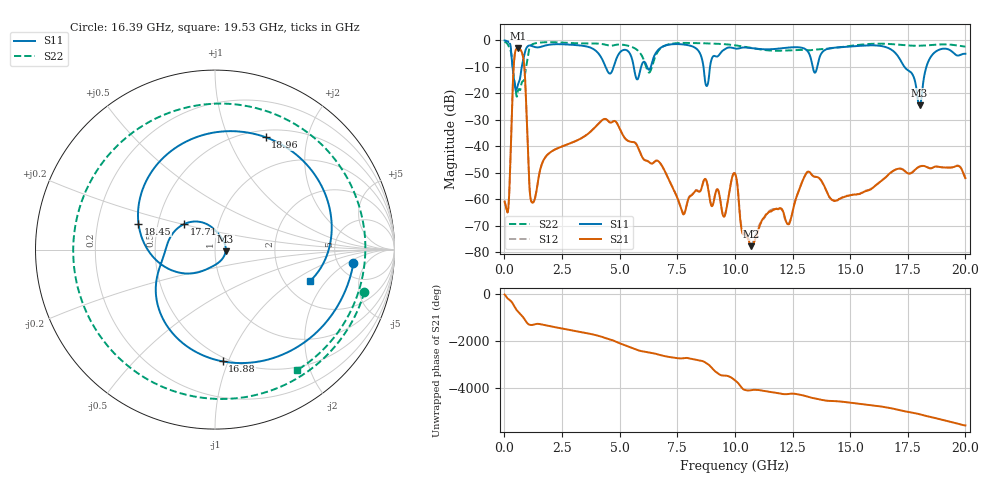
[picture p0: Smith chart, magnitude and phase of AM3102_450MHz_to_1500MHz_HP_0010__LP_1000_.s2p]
!Agilent Technologies,E8364B,MY43040894,A.07.50.67
!Agilent E8364B: A.07.50.67
!Date: Thursday, January 11, 2018 05:27:46
!Correction: S11(Full 2 Port(1,2))
!S21(Full 2 Port(1,2))
!S12(Full 2 Port(1,2))
!S22(Full 2 Port(1,2))
!S2P File: Measurements: S11, S21, S12, S22:
# Hz S  dB  R 50
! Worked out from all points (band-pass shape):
!   1601 points, 10 MHz to 20 GHz, reference 50 ohm
!   highest |S21| = -3.07 dB at 584.7 MHz (marker M1); lowest = -77.7 dB at 10.7 GHz (marker M2)
!   |S21| within 3 dB of the highest: 440.4 MHz to 805.1 MHz (364.7 MHz wide, 58.6 % of centre)
!   lowest |S11| = -24.5 dB at 18.01 GHz (marker M3), VSWR 1.13, Z = 56.2 - j1.17 ohm
!   |S11| at or under -10 dB: 355.2 MHz to 754.6 MHz (399.4 MHz wide, 72 % of centre); 4.39 GHz to 4.741 GHz (351 MHz wide, 7.69 % of centre); 17.35 GHz to 18.31 GHz (953.1 MHz wide, 5.35 % of centre)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
!   |S22| runs from -21.2 to -0.5 dB; largest |S21 - S12| = 0.0016
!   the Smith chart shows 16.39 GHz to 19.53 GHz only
!   S11 on the Smith chart (normalised r, x): 16.39 GHz: 6.94, -2.54; 16.88 GHz: 0.47, -0.95; 17.71 GHz: 0.68, +0.20; 18.45 GHz: 0.39, +0.14; 18.96 GHz: 0.58, +1.38; 19.53 GHz: 2.75, -1.39
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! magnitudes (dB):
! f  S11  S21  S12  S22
! 10 MHz  -0.1  -60.9  -60.5  -0.5
! 172.4 MHz  -0.6  -63.2  -63.0  -2.0
! 409.8 MHz  -14.2  -9.2  -9.2  -14.0
! 584.7 MHz  -16.9  -3.1  -3.1  -19.1
! 834.6 MHz  -6.7  -7.5  -7.5  -15.3
! 1.209 GHz  -2.2  -61.2  -61.0  -1.5
! 3.346 GHz  -2.0  -36.9  -36.9  -1.2
! 6.682 GHz  -3.5  -45.6  -45.6  -4.0
! 7.769 GHz  -1.6  -65.7  -65.2  -1.0
! 8.781 GHz  -17.3  -53.4  -53.4  -1.2
! 10.01 GHz  -3.1  -50.3  -50.3  -1.9
! 10.7 GHz  -2.9  -77.7  -77.2  -2.9
! 13.34 GHz  -8.6  -50.8  -50.7  -3.7
! 16.39 GHz  -2.2  -52.8  -52.7  -1.3
! 16.68 GHz  -3.0  -50.5  -50.5  -1.4
! 16.88 GHz  -4.1  -49.2  -49.2  -1.5
! 17.71 GHz  -13.0  -49.7  -49.6  -2.0
! 18.01 GHz  -24.5  -47.7  -47.6  -2.0
! 18.45 GHz  -6.9  -48.3  -48.2  -1.8
! 18.96 GHz  -3.3  -47.9  -47.9  -1.5
! 19.53 GHz  -5.1  -47.7  -47.6  -1.8
! 20 GHz  -5.1  -52.0  -52.1  -2.4
